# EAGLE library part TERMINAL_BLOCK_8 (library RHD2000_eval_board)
8-point terminal block
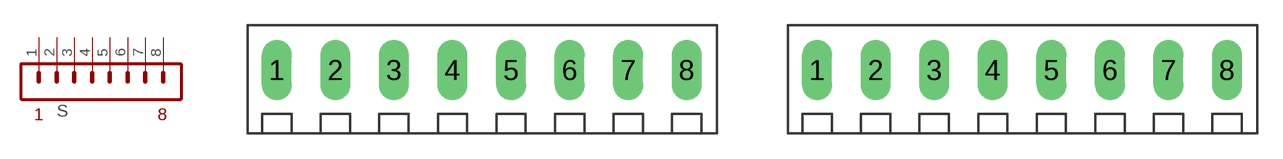
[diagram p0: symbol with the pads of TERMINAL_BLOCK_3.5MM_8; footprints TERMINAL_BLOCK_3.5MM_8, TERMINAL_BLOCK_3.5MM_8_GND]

Designator prefix S

## TERMINAL_BLOCK_8-3.5MM  [TERMINAL_BLOCK_3.5MM_8]
1  1  pas
2  2  pas
3  3  pas
4  4  pas
5  5  pas
6  6  pas
7  7  pas
8  8  pas

## TERMINAL_BLOCK_8-3.5MM-GND  [TERMINAL_BLOCK_3.5MM_8_GND]
Pads as for TERMINAL_BLOCK_3.5MM_8

## Footprint TERMINAL_BLOCK_3.5MM_8 (pad centres in mm)
drill 1.2 long: 1 -12.28,0; 2 -8.78,0; 3 -5.28,0; 4 -1.78,0; 5 1.72,0; 6 5.22,0; 7 8.72,0; 8 12.22,0

## Footprint TERMINAL_BLOCK_3.5MM_8_GND (pad centres in mm)
drill 1.2 long: 1 -12.28,0; 2 -8.78,0; 3 -5.28,0; 4 -1.78,0; 5 1.72,0; 6 5.22,0; 7 8.72,0; 8 12.22,0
